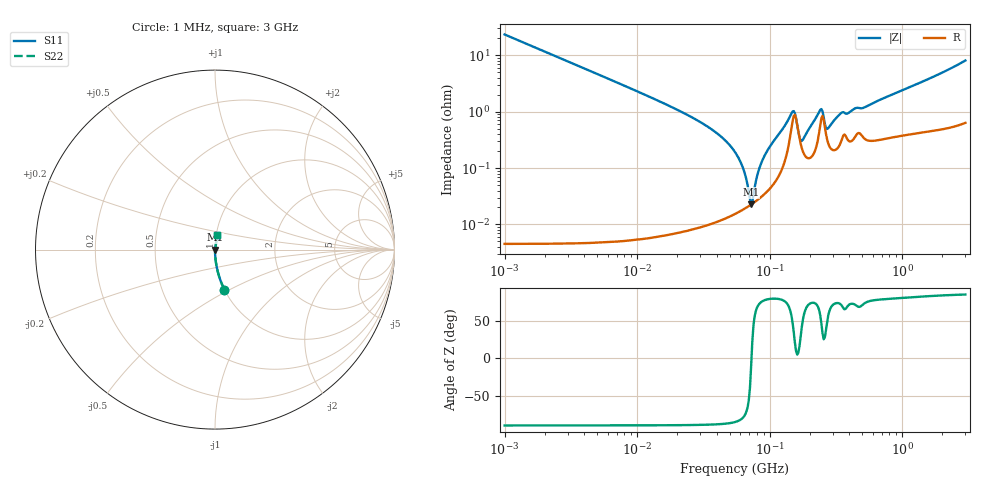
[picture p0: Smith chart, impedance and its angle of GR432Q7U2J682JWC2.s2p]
!Murata Part Number: GR432Q7U2J682JWC2
!These Parameters are Measured in Series Mode Connection
!Data Generated on Jun 10, 2025
!  o--ll--o
!Port1  Port2
!  o------o
!Operation Temp=25[degC], DC Bias Voltage=0[V]
!Freq. Start=1000[kHz] Stop=3[GHz] 401[Steps]
# Hz S RI R 50
!Freq.(Hz) S11(Real) S11(Imag) S21(Real) S21(Imag) S12(Real) S12(Imag) S22(Real) S22(Imag)
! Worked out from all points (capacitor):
!   401 points, 1 MHz to 3 GHz, reference 50 ohm
!   read as one part in series: C = 6.77 nF near 1.041 MHz
!   lowest |Z| = 23 mohm at 72.49 MHz (marker M1)
!   series resonance near 72.95 MHz, so ESL is about 700 pH
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1000000  0.0524 -0.2226  0.9476 0.2226  0.9476 0.2226  0.0524 -0.2226
3823119  0.00379 -0.0611  0.9962 0.0611  0.9962 0.0611  0.00379 -0.0611
1.461624e7  0.000299 -0.0154  0.9997 0.0154  0.9997 0.0154  0.000299 -0.0154
3.526298e7  0.000126 -0.00515  0.9999 0.00515  0.9999 0.00515  0.000126 -0.00515
5.477226e7  0.000157 -0.00192  0.9998 0.00192  0.9998 0.00192  0.000157 -0.00192
6.301011e7  0.000184 -0.00098  0.9998 0.00098  0.9998 0.00098  0.000184 -0.00098
7.248696e7  0.000226 -4.26e-05  0.9998 4.26e-05  0.9998 4.26e-05  0.000226 -4.26e-05
7.544761e7  0.000241 0.00023  0.9998 -0.00023  0.9998 -0.00023  0.000241 0.00023
8.173662e7  0.000277 0.000787  0.9997 -0.000787  0.9997 -0.000787  0.000277 0.000787
9.034013e7  0.00034 0.00152  0.9997 -0.00152  0.9997 -0.00152  0.00034 0.00152
1.460522e8  0.0051 0.00778  0.9949 -0.00778  0.9949 -0.00778  0.0051 0.00778
1.550909e8  0.00873 0.0033  0.9913 -0.0033  0.9913 -0.0033  0.00873 0.0033
1.680187e8  0.00335 0.000986  0.9967 -0.000986  0.9967 -0.000986  0.00335 0.000986
1.748812e8  0.00225 0.00203  0.9977 -0.00203  0.9977 -0.00203  0.00225 0.00203
2.094008e8  0.00166 0.00585  0.9983 -0.00585  0.9983 -0.00585  0.00166 0.00585
2.408952e8  0.00583 0.00902  0.9942 -0.00902  0.9942 -0.00902  0.00583 0.00902
2.507343e8  0.00844 0.00549  0.9916 -0.00549  0.9916 -0.00549  0.00844 0.00549
2.662515e8  0.00401 0.00317  0.996 -0.00317  0.996 -0.00317  0.00401 0.00317
2.771263e8  0.00272 0.00433  0.9973 -0.00433  0.9973 -0.00433  0.00272 0.00433
3.453811e8  0.00299 0.00892  0.997 -0.00892  0.997 -0.00892  0.00299 0.00892
8.005644e8  0.00376 0.0188  0.9962 -0.0188  0.9962 -0.0188  0.00376 0.0188
3e9  0.0127 0.0794  0.9873 -0.0794  0.9873 -0.0794  0.0127 0.0794
